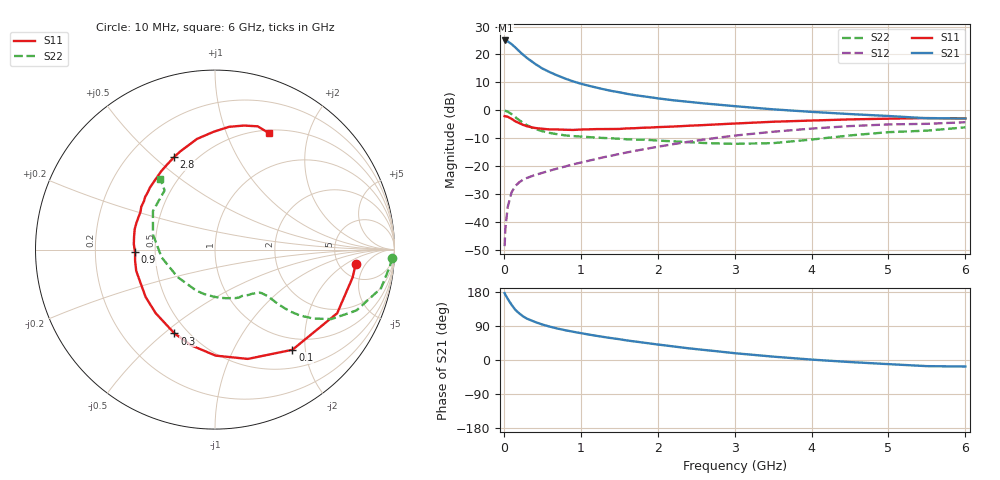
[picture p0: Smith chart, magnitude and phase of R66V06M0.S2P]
! SIEMENS Small Signal Semiconductors
! BFR193
! Si NPN RF Bipolar Junction Transistor in SOT23
! VCE = 6 V  IC = 6 mA
! Common Emitter S-Parameters:  May  1996
# GHz  S  MA  R  50
!  f  S11  S21  S12  S22
! GHz  MAG  ANG  MAG  ANG  MAG  ANG  MAG  ANG
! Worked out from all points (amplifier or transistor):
!   36 points, 10 MHz to 6 GHz, reference 50 ohm
!   highest |S21| = 25.0 dB at 20 MHz (marker M1)
!   |S21| within 3 dB of that: start of sweep to 168.1 MHz
!   unconditionally stable (mu >= 1): 857.5 MHz to 2.009 GHz
!   at 250 MHz: K = 0.47, MSG = 22.4 dB, |S12| = -24.8 dB
!   at 1.4 GHz: K = 1.06, MAG = 10.1 dB, |S12| = -16.2 dB
!   at 6 GHz: K = 0.95, MSG = 0.7 dB, |S12| = -4.3 dB
!   lowest NFmin = 1.20 dB at 450 MHz
!   S11 on the Smith chart (normalised r, x): 10 MHz: 7.19, -2.97; 100 MHz: 0.79, -1.76; 300 MHz: 0.42, -0.54; 900 MHz: 0.38, -0.01; 2.8 GHz: 0.39, +0.58; 6 GHz: 0.53, +1.42
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0.01  0.7881 -5.7  17.67 176.4  0.0037 86.7  0.9888 -2.6
0.02  0.7824 -11.4  17.84 172.2  0.0077 83.7  0.9793 -5.4
0.05  0.7675 -27.5  17.16 161.5  0.0185 77.3  0.9496 -13.1
0.1  0.7054 -52.3  15.36 145.8  0.0339 66.1  0.8577 -23.3
0.15  0.6359 -73.3  13.34 132.3  0.0443 58.5  0.7541 -30.9
0.2  0.5906 -89.7  11.46 123.0  0.0515 53.9  0.6679 -35.1
0.25  0.5497 -103.9  9.895 115.2  0.0573 51.5  0.5981 -37.8
0.3  0.5187 -115.8  8.686 109.2  0.0616 50.6  0.5415 -39.5
0.4  0.4845 -133.0  6.889 100.8  0.0692 50.0  0.4684 -40.8
0.5  0.4683 -145.6  5.622 93.7  0.076 50.8  0.4231 -41.1
0.6  0.4545 -156.0  4.809 87.9  0.0835 52.2  0.3932 -41.5
0.7  0.4547 -164.9  4.191 82.8  0.0912 54.0  0.3725 -42.2
0.9  0.4457 -178.1  3.303 74.6  0.1078 56.3  0.3462 -43.9
1.1  0.4567 170.9  2.764 67.3  0.125 58.2  0.3323 -47.0
1.3  0.4624 161.3  2.38 60.7  0.145 59.3  0.3198 -50.5
1.6  0.4752 149.8  1.979 51.6  0.1765 59.7  0.3031 -57.8
2.2  0.5124 130.4  1.516 35.9  0.2478 56.7  0.2787 -76.5
2.8  0.5631 113.9  1.259 22.4  0.326 50.3  0.2551 -103.4
3.5  0.6249 99.2  1.043 8.9  0.4137 40.0  0.2588 -144.0
4.5  0.6885 83.5  0.858 -5.4  0.5227 24.0  0.3556 166.4
5.5  0.727 70.9  0.722 -16.2  0.5738 7.2  0.4331 130.4
6  0.7153 65.3  0.715 -17.2  0.6127 2.4  0.496 127.8
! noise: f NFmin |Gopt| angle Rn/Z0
0.45  1.2  0.25  114  0.13
0.9  1.25  0.37  150  0.12
1.8  2  0.55  -158  0.12
